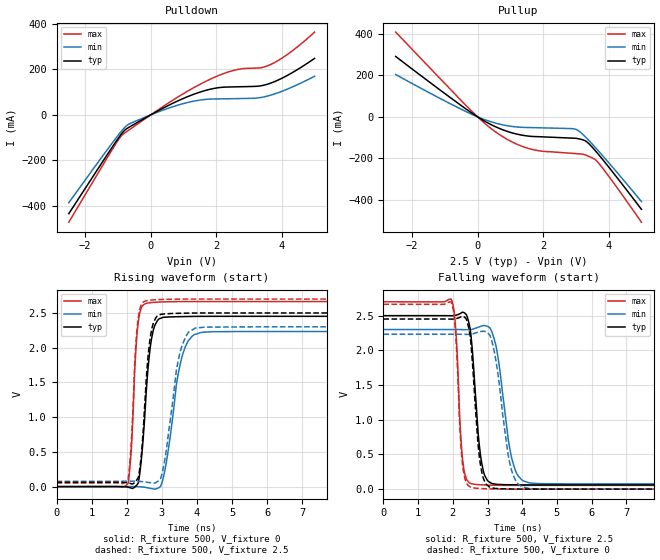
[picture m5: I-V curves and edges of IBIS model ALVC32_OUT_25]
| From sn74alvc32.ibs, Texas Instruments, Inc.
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[Model]   ALVC32_OUT_25
Model_type  Output
Vref =   0
Rref =   500
Cref =   30p
Vmeas =   1.25
| variable   typ   min   max
C_comp   7.89pF   5.59pF   10.52pF
| C_pullup   8.52pF   6.52pF   10.21pF
| C_pulldown   7.27pF   5.59pF   10.52pF
[Temperature Range]   40   100   -40
| Ambient temperature   25   85   -40
[Voltage range]   2.5   2.3   2.7
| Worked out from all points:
|   slope of the pulldown table from 0 to 0.375 V, typ, clamps not added: 12.8 ohm
|   slope of the pullup table from 0 to 0.375 V, typ, clamps not added: 10.9 ohm
|   rising waveform, R_fixture 500, V_fixture 0: 20-80 % time 224ps typ, 375ps min, 153ps max; typ from 0 V to 2.45 V
|   falling waveform, R_fixture 500, V_fixture 2.5: 20-80 % time 222ps typ, 351ps min, 151ps max; typ from 2.5 V to 0.061 V
|   rising waveform, R_fixture 500, V_fixture 2.5: 20-80 % time 205ps typ, 359ps min, 154ps max; typ from 0.061 V to 2.5 V
|   falling waveform, R_fixture 500, V_fixture 0: 20-80 % time 215ps typ, 349ps min, 153ps max; typ from 2.45 V to 0 V
[Pulldown]
| ALVC32_OUT_25
|   Voltage   I(typ)   I(min)   I(max)
-2.5V     -433.6mA   -385.5mA   -471mA
-1.045V   -114.1mA   -98.92mA   -122.1mA
-890mV    -83.15mA   -70.84mA   -91.01mA
-715mV    -59.03mA   -45.2mA    -71.58mA
735mV     55.03mA    38.42mA    69.88mA
1.325V    90.9mA     60.41mA    120.2mA
1.83V     112.9mA    69.33mA    157.4mA
2.53V     122.7mA    70.94mA    195mA
3.37V     127.6mA    76.43mA    206.9mA
3.775V    145.6mA    91.54mA    229.3mA
4.32V     185.2mA    122.2mA    280.8mA
5V        247.8mA    169.5mA    363.1mA
[Pullup]
| ALVC32_OUT_25
|   Voltage   I(typ)   I(min)   I(max)
-2.5V     290.4mA    203.5mA    407.5mA
-235mV    24.72mA    16.51mA    35.93mA
230mV     -22mA      -14.22mA   -32.72mA
660mV     -55.34mA   -34.57mA   -84.31mA
1.155V    -81.27mA   -48.01mA   -128.3mA
1.655V    -93.93mA   -51.65mA   -156.2mA
2.85V     -102mA     -56.39mA   -174.9mA
3.035V    -104mA     -62.79mA   -177.1mA
3.315V    -118.2mA   -100.4mA   -184.6mA
3.645V    -172.4mA   -156.5mA   -214mA
4.1V      -260.8mA   -238.6mA   -306.6mA
5V        -444.6mA   -407.2mA   -506.3mA
[Ramp]
| ALVC32_OUT_25
| variable   typ   min   max
dV/dt_r   1.49/2.50E-10   1.36/4.18E-10   1.60/1.56E-10
dV/dt_f   1.49/2.36E-10   1.37/3.85E-10   1.61/1.60E-10
R_load = 500
[Rising Waveform]
| ALVC32_OUT_25
R_fixture =   500
C_fixture =   0
L_fixture =   0
V_fixture =   0
V_fixture_min = 0
V_fixture_max = 0
|   Time   V(typ)   V(min)   V(max)
0s        34.48pV    4.63nV     26.61pV
2.04ns    -8.926mV   1.081mV    48.88mV
2.13ns    -21.73mV   1.235mV    537.3mV
2.235ns   -4.332mV   1.185mV    1.755V
2.33ns    53.52mV    -1.14mV    2.375V
2.71ns    2.14V      -28.74mV   2.651V
3.05ns    2.438V     147.8mV    2.66V
3.61ns    2.448V     1.93V      2.664V
4.17ns    2.451V     2.223V     2.664V
50ns      2.451V     2.232V     2.664V
[Falling Waveform]
| ALVC32_OUT_25
R_fixture =   500
C_fixture =   0
L_fixture =   0
V_fixture =   2.5
V_fixture_min = 2.3
V_fixture_max = 2.7
|   Time   V(typ)   V(min)   V(max)
0s        2.5V       2.3V       2.7V
1.955ns   2.499V     2.3V       2.737V
2.085ns   2.506V     2.3V       2.297V
2.305ns   2.547V     2.299V     332.8mV
2.5ns     2.311V     2.298V     85.34mV
2.685ns   1.131V     2.325V     66.05mV
2.995ns   126.5mV    2.347V     57.64mV
3.73ns    61.82mV    383.5mV    53.08mV
4.24ns    60.11mV    87.59mV    53mV
50ns      60.54mV    76.61mV    53.33mV
[Rising Waveform]
| ALVC32_OUT_25
R_fixture =   500
C_fixture =   0
L_fixture =   0
V_fixture =   2.5
V_fixture_min = 2.3
V_fixture_max = 2.7
|   Time   V(typ)   V(min)   V(max)
0s        60.54mV    76.61mV    53.33mV
2.04ns    52.33mV    77.5mV     109mV
2.13ns    41.29mV    77.57mV    640.2mV
2.23ns    62.02mV    77.5mV     1.805V
2.325ns   127.6mV    75.47mV    2.421V
2.7ns     2.235V     54.1mV     2.687V
3.025ns   2.482V     231mV      2.695V
3.55ns    2.496V     1.991V     2.699V
4.015ns   2.499V     2.29V      2.7V
50ns      2.5V       2.3V       2.7V
[Falling Waveform]
| ALVC32_OUT_25
R_fixture =   500
C_fixture =   0
L_fixture =   0
V_fixture =   0
V_fixture_min = 0
V_fixture_max = 0
|   Time   V(typ)   V(min)   V(max)
0s        2.451V     2.232V     2.664V
1.955ns   2.45V      2.232V     2.695V
2.075ns   2.456V     2.232V     2.281V
2.29ns    2.493V     2.231V     314mV
2.5ns     2.209V     2.231V     32.55mV
2.69ns    895.9mV    2.256V     12.08mV
2.97ns    65.03mV    2.26V      4.435mV
3.685ns   1.084mV    285.6mV    -169.4uV
4.21ns    -343.4uV   7.975mV    -315.3uV
50ns      35.08pV    4.63nV     26.43pV
